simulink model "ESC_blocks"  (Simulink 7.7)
settings: Solver=ode45  StartTime=0.0  StopTime=10.0  RelTol=1e-3
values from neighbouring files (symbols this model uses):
  stepsize = 0.001    [sim_run_multi.m]    (also in sim_run_uni.m)
  x0 = [0;0]    [sim_run_multi.m]    (also in sim_run_uni.m = 0)
undefined symbols (not defined in the file or in its folder): adaptive_sampling, approx, nn, perturb, sm_periodic, vel_init_adap

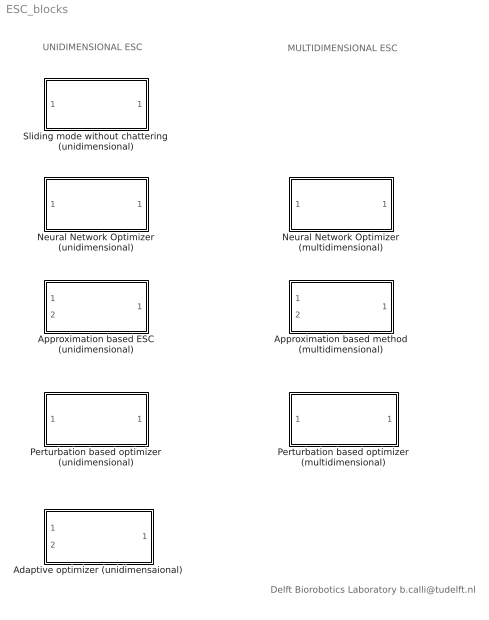
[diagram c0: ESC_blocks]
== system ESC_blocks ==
  note: UNIDIMENSIONAL ESC
  note: MULTIDIMENSIONAL ESC
  note: Delft Biorobotics Laboratory b.calli@tudelft.nl
  Adaptive optimizer (unidimensaional) : Subsystem  mask{adaptive_sampling=adaptive_sampling, vel_init=vel_init_adap, stepsize=stepsize, data_size=10, x0=x0}
      mask prompts: adaptive_sampling "Sampling (cycle)"; vel_init "Initial Velocity (while collecting initial data points)"; stepsize "Step size"; data_size "Data size"; x0 "Initial position"
  Approximation based ESC (unidimensional) : Subsystem  mask{K_grad=approx.K_grad, sampling=approx.sampling, data_size=approx.data_size, poly_degree=approx.poly_degree, vel_init=approx.vel_init, lpf_constant=approx.filter_constant}
      mask prompts: data_size "Data size"; poly_degree "Poly degree"; vel_init "Initial velocity"; lpf_constant "Filter Constant"
  Approximation based method (multidimensional) : Subsystem  mask{K_grad=approx.K_grad, sampling=approx.sampling, data_size=approx.data_size, vel_init=approx.vel_init, lpf_constant=approx.filter_constant}
      mask prompts: K_grad "Gain"; data_size "Data size"; vel_init "Initial velocity"; lpf_constant "Low pass filter constant"
  Neural Network Optimizer (multidimensional) : Subsystem  mask{M=nn.M, A=nn.A, B=nn.B, ddelta1=nn.ddelta1, ddelta2=nn.ddelta2, ddelta3=nn.ddelta3, delta=nn.delta, mpd_init=nn.mpd_init}
      mask prompts: ddelta1 "Direction 1 delta"; ddelta2 "Direction 2 delta"; ddelta3 "Direction 3 delta"; mpd_init "Minimum Peak Detector initial value"
  Neural Network Optimizer (unidimensional) : Subsystem  mask{M=nn.M, A=nn.A, B=nn.B, ddelta=nn.ddelta, delta=nn.delta, mpd_init=nn.mpd_init}
      mask prompts: mpd_init "Minimum peak detector initial value"
  Perturbation based optimizer (multidimensional) : Subsystem  mask{corr_gain=perturb.corr_gain, low_pass_pole=perturb.low_pass_pole, high_pass_pole=perturb.high_pass_pole, sine_amp=perturb.sine_amp, sine_freq=perturb.sine_freq, sine_phase=perturb.sine_phase, comp_zero=perturb.comp_zero, comp_pole=perturb.comp_pole}
      mask prompts: corr_gain "Correction gain"; low_pass_pole "Low Pass Filter pole"; high_pass_pole "High Pass Filter pole"; sine_amp "Sinus amplitude"; sine_freq "Sinus frequency"; sine_phase "Sinus phase"; comp_zero "Compensator zero"; comp_pole "Compensator pole"
  Perturbation based optimizer (unidimensional) : Subsystem  mask{high_pass_pole=perturb.high_pass_pole, sine_amp=perturb.sine_amp, sine_freq=perturb.sine_freq, low_pass_pole=perturb.low_pass_pole, corr_gain=perturb.corr_gain, comp_zero=perturb.comp_zero, comp_pole=perturb.comp_pole}
      mask prompts: high_pass_pole "High Pass Filter Pole"; sine_amp "Perturbation Signal Amplitude"; sine_freq "Perturbation Signal Frequency"; low_pass_pole "Low Pass Filter Pole"; corr_gain "Correction Gain"; comp_zero "Compensator Zero"; comp_pole "Compensator Pole"
  Sliding mode without chattering (unidimensional) : Subsystem  mask{alpha=sm_periodic.alpha, rho=sm_periodic.rho, k=sm_periodic.k, g_init=sm_periodic.g_init}
      mask prompts: g_init "initial g"

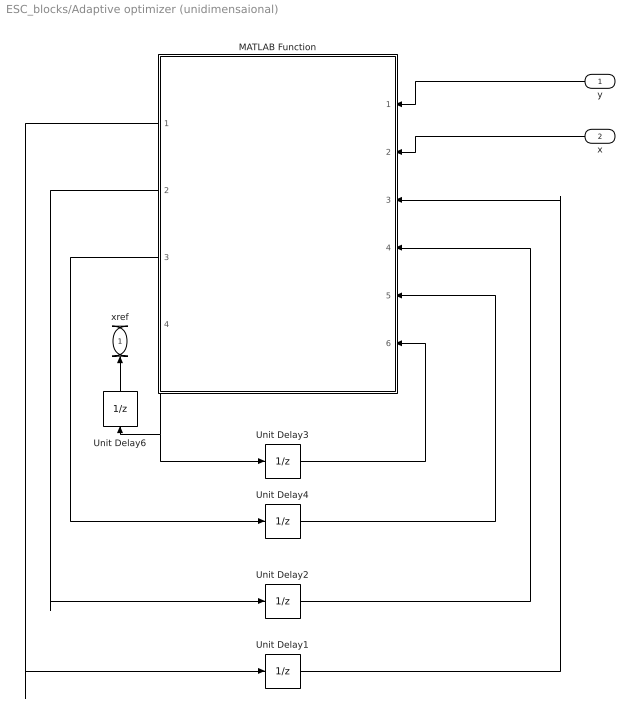
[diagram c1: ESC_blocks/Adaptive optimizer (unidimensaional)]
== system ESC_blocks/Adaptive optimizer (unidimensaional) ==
  y : Inport
  x : Inport  Port=2
  MATLAB Function : Stateflow chart  TreatAsAtomicUnit=on
  Unit Delay1 : UnitDelay  SampleTime=-1
  Unit Delay2 : UnitDelay  X0=zeros(data_size,3)  SampleTime=-1
  Unit Delay3 : UnitDelay  SampleTime=-1
  Unit Delay4 : UnitDelay  X0=zeros(data_size,1)  SampleTime=-1
  Unit Delay6 : UnitDelay  X0=x0  SampleTime=-1
  xref : Outport
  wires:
  y/1 -> MATLAB Function/1(y_data_in)
  MATLAB Function/4(x_ref) -> Unit Delay3/1, Unit Delay6/1
  Unit Delay3/1 -> MATLAB Function/6(x_ref_in)
  MATLAB Function/1(sample_out) -> Unit Delay1/1
  Unit Delay1/1 -> MATLAB Function/3(sample)
  MATLAB Function/2(phi_data_out) -> Unit Delay2/1
  MATLAB Function/3(y_array_out) -> Unit Delay4/1
  Unit Delay4/1 -> MATLAB Function/5(y_array)
  Unit Delay6/1 -> xref/1
  Unit Delay2/1 -> MATLAB Function/4(phi_data)
  x/1 -> MATLAB Function/2(x_in)

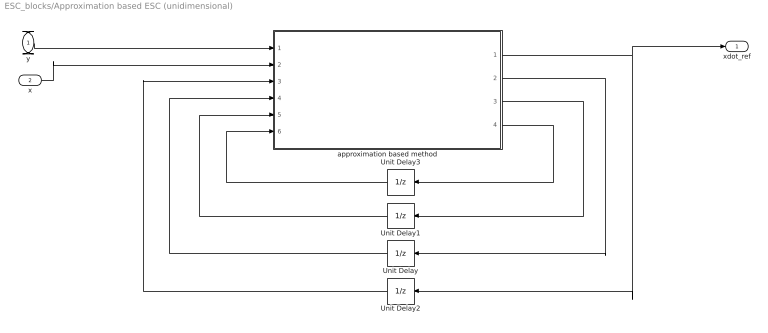
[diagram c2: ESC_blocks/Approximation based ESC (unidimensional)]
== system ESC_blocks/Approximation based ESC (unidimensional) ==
  y : Inport
  x : Inport  Port=2
  Unit Delay : UnitDelay  X0=zeros(1,data_size)  SampleTime=-1
  Unit Delay1 : UnitDelay  X0=zeros(1,data_size)  SampleTime=-1
  Unit Delay2 : UnitDelay  SampleTime=-1
  Unit Delay3 : UnitDelay  SampleTime=-1
  approximation based method : Stateflow chart  TreatAsAtomicUnit=on
  xdot_ref : Outport
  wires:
  approximation based method/2(x_data_arr_out) -> Unit Delay/1
  Unit Delay/1 -> approximation based method/4(x_data_arr)
  approximation based method/3(y_data_arr_out) -> Unit Delay1/1
  Unit Delay1/1 -> approximation based method/5(y_data_arr)
  y/1 -> approximation based method/1(y_data_in)
  x/1 -> approximation based method/2(x_data_in)
  approximation based method/1(xdot_ref) -> Unit Delay2/1, xdot_ref/1
  approximation based method/4(sample_out) -> Unit Delay3/1
  Unit Delay2/1 -> approximation based method/3(xdot_ref_in)
  Unit Delay3/1 -> approximation based method/6(sample)

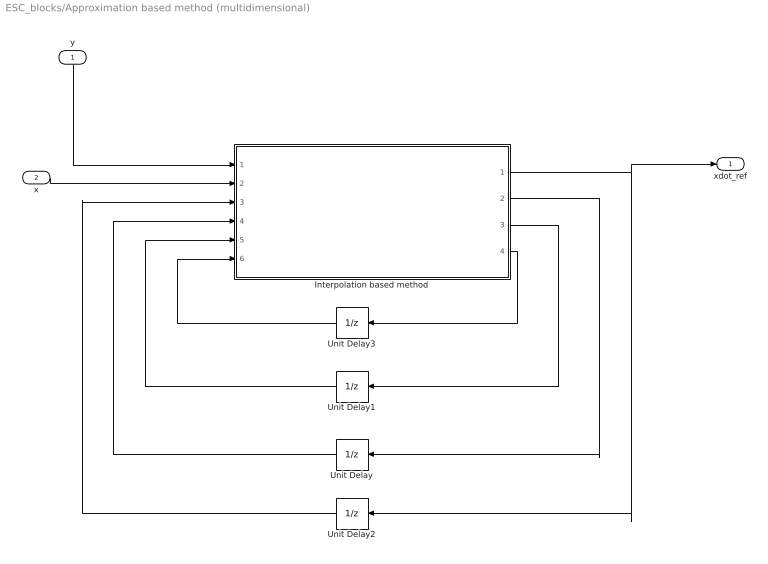
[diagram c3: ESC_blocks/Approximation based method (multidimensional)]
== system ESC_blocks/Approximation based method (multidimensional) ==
  y : Inport
  x : Inport  Port=2
  Interpolation based method : Stateflow chart  TreatAsAtomicUnit=on
  Unit Delay : UnitDelay  X0=[zeros(1,data_size);zeros(1,data_size)]  SampleTime=-1
  Unit Delay1 : UnitDelay  X0=zeros(1,data_size)  SampleTime=-1
  Unit Delay2 : UnitDelay  X0=[0;0]  SampleTime=-1
  Unit Delay3 : UnitDelay  SampleTime=-1
  xdot_ref : Outport
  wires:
  Unit Delay/1 -> Interpolation based method/4(x_data)
  Unit Delay1/1 -> Interpolation based method/5(y_data)
  y/1 -> Interpolation based method/1(y_data_in)
  x/1 -> Interpolation based method/2(x_data_in)
  Unit Delay2/1 -> Interpolation based method/3(xdot_ref_in)
  Unit Delay3/1 -> Interpolation based method/6(sample)
  Interpolation based method/4(sample_out) -> Unit Delay3/1
  Interpolation based method/3(y_data_out) -> Unit Delay1/1
  Interpolation based method/2(x_data_out) -> Unit Delay/1
  Interpolation based method/1(xdot_ref) -> Unit Delay2/1, xdot_ref/1

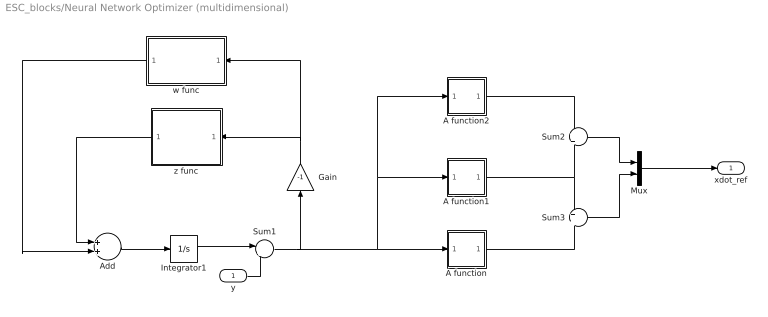
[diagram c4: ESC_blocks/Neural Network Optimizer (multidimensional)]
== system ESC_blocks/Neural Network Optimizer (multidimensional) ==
  y : Inport
  A function : Subsystem
  A function1 : Subsystem
  A function2 : Subsystem
  Add : Sum
  Gain : Gain  Gain=-1
  Integrator1 : Integrator  InitialCondition=mpd_init
  Mux : Mux  Inputs=2
  Sum1 : Sum  Inputs=|+-
  Sum2 : Sum  Inputs=+|+
  Sum3 : Sum  Inputs=+|+
  w func : Subsystem
  z func : Subsystem
  xdot_ref : Outport
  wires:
  Sum1/1 -> Gain/1, A function/1(e), A function1/1(e), A function2/1(e)
  Gain/1 -> w func/1(e_minus), z func/1(e_minus)
  w func/1(w) -> Add/2
  z func/1(z) -> Add/1
  Add/1 -> Integrator1/1
  Integrator1/1 -> Sum1/1
  A function2/1(xdot) -> Sum2/1
  A function1/1(xdot) -> Sum2/2, Sum3/1
  A function/1(xdot) -> Sum3/2
  Sum2/1 -> Mux/1
  Sum3/1 -> Mux/2
  Mux/1 -> xdot_ref/1
  y/1 -> Sum1/2

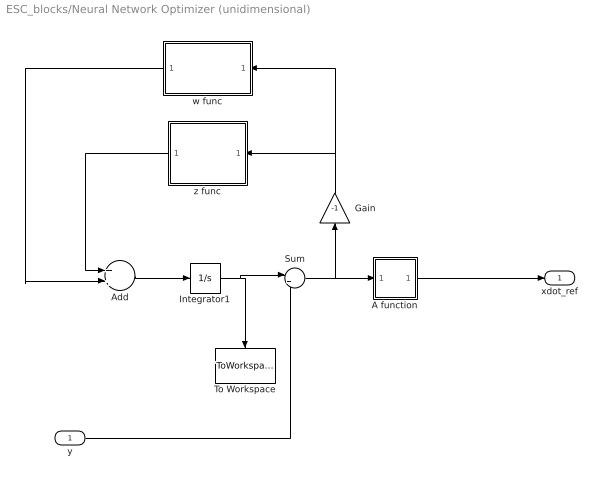
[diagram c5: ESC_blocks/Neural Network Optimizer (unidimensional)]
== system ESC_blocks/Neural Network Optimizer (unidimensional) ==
  y : Inport
  A function : Subsystem
  Add : Sum
  Gain : Gain  Gain=-1
  Integrator1 : Integrator  InitialCondition=mpd_init
  Sum : Sum  Inputs=|+-
  To Workspace : ToWorkspace  VariableName=yd_out  SampleTime=-1  SaveFormat=Structure With Time
  w func : Subsystem
  z func : Subsystem
  xdot_ref : Outport
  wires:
  Sum/1 -> Gain/1, A function/1(e)
  Gain/1 -> w func/1(e_minus), z func/1(e_minus)
  w func/1(w) -> Add/2
  z func/1(z) -> Add/1
  Add/1 -> Integrator1/1
  Integrator1/1 -> Sum/1, To Workspace/1
  A function/1(xdot) -> xdot_ref/1
  y/1 -> Sum/2

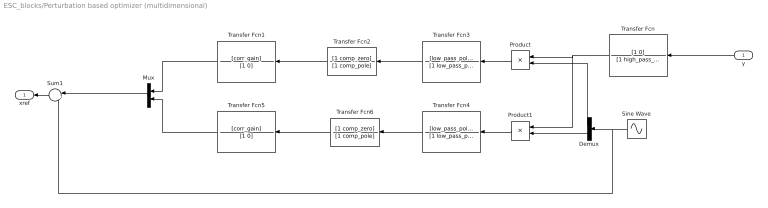
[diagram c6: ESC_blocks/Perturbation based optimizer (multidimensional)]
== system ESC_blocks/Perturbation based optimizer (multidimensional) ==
  y : Inport
  Demux : Demux  Outputs=2
  Mux : Mux  Inputs=2
  Product : Product  Multiplication=Matrix(*)
  Product1 : Product  Multiplication=Matrix(*)
  Sine Wave : Sin  Amplitude=[sine_amp sine_amp]  Frequency=[sine_freq sine_freq]  Phase=[0 sine_phase]  SampleTime=0
  Sum1 : Sum  Inputs=|++
  Transfer Fcn : TransferFcn  Numerator=[1 0]  Denominator=[1 high_pass_pole]
  Transfer Fcn1 : TransferFcn  Numerator=[corr_gain]  Denominator=[1 0]
  Transfer Fcn2 : TransferFcn  Numerator=[1 comp_zero]  Denominator=[1 comp_pole]
  Transfer Fcn3 : TransferFcn  Numerator=[low_pass_pole]  Denominator=[1 low_pass_pole]
  Transfer Fcn4 : TransferFcn  Numerator=[low_pass_pole]  Denominator=[1 low_pass_pole]
  Transfer Fcn5 : TransferFcn  Numerator=[corr_gain]  Denominator=[1 0]
  Transfer Fcn6 : TransferFcn  Numerator=[1 comp_zero]  Denominator=[1 comp_pole]
  xref : Outport
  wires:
  y/1 -> Transfer Fcn/1
  Sum1/1 -> xref/1
  Transfer Fcn/1 -> Product/1, Product1/1
  Sine Wave/1 -> Demux/1, Sum1/2
  Demux/1 -> Product/2
  Demux/2 -> Product1/2
  Product/1 -> Transfer Fcn3/1
  Product1/1 -> Transfer Fcn4/1
  Transfer Fcn3/1 -> Transfer Fcn2/1
  Transfer Fcn4/1 -> Transfer Fcn6/1
  Transfer Fcn1/1 -> Mux/1
  Transfer Fcn5/1 -> Mux/2
  Mux/1 -> Sum1/1
  Transfer Fcn2/1 -> Transfer Fcn1/1
  Transfer Fcn6/1 -> Transfer Fcn5/1

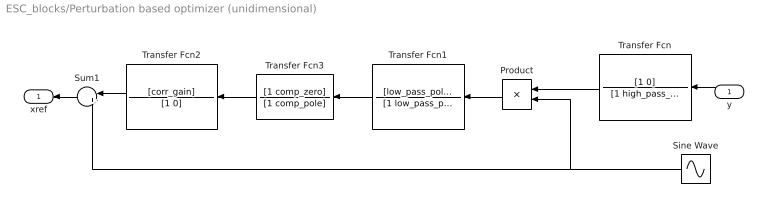
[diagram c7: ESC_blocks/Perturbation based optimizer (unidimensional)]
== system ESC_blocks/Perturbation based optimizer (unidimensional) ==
  y : Inport
  Product : Product
  Sine Wave : Sin  Amplitude=sine_amp  Frequency=sine_freq  SampleTime=0
  Sum1 : Sum  Inputs=|++
  Transfer Fcn : TransferFcn  Numerator=[1 0]  Denominator=[1 high_pass_pole]
  Transfer Fcn1 : TransferFcn  Numerator=[low_pass_pole]  Denominator=[1 low_pass_pole]
  Transfer Fcn2 : TransferFcn  Numerator=[corr_gain]  Denominator=[1 0]
  Transfer Fcn3 : TransferFcn  Numerator=[1 comp_zero]  Denominator=[1 comp_pole]
  xref : Outport
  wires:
  Transfer Fcn/1 -> Product/1
  Sine Wave/1 -> Product/2, Sum1/2
  Product/1 -> Transfer Fcn1/1
  Transfer Fcn1/1 -> Transfer Fcn3/1
  Transfer Fcn2/1 -> Sum1/1
  y/1 -> Transfer Fcn/1
  Sum1/1 -> xref/1
  Transfer Fcn3/1 -> Transfer Fcn2/1

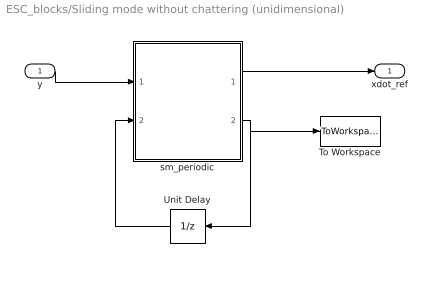
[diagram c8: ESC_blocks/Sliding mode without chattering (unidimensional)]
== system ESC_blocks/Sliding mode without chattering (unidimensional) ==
  y : Inport
  To Workspace : ToWorkspace  VariableName=g_sm_out  SampleTime=-1  SaveFormat=Structure With Time
  Unit Delay : UnitDelay  X0=g_init  SampleTime=-1
  sm_periodic : Stateflow chart  TreatAsAtomicUnit=on
  xdot_ref : Outport
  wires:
  y/1 -> sm_periodic/1(y)
  sm_periodic/1(u) -> xdot_ref/1
  sm_periodic/2(g_out) -> Unit Delay/1, To Workspace/1
  Unit Delay/1 -> sm_periodic/2(g_in)

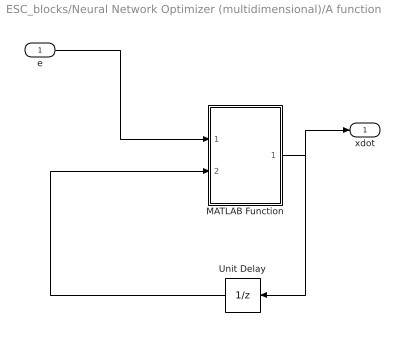
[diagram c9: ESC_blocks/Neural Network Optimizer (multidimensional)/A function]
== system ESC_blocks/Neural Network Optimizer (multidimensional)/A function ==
  e : Inport
  MATLAB Function : Stateflow chart  TreatAsAtomicUnit=on
  Unit Delay : UnitDelay  X0=A  SampleTime=-1
  xdot : Outport
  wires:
  Unit Delay/1 -> MATLAB Function/2(state_pre)
  MATLAB Function/1(xdot) -> xdot/1, Unit Delay/1
  e/1 -> MATLAB Function/1(e)

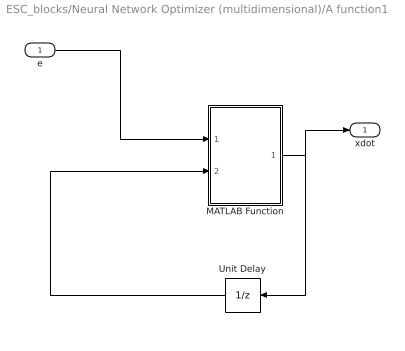
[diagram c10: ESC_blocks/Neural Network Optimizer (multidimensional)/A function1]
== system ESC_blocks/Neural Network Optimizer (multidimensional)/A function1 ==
  e : Inport
  MATLAB Function : Stateflow chart  TreatAsAtomicUnit=on
  Unit Delay : UnitDelay  SampleTime=-1
  xdot : Outport
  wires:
  e/1 -> MATLAB Function/1(e)
  MATLAB Function/1(xdot) -> Unit Delay/1, xdot/1
  Unit Delay/1 -> MATLAB Function/2(state_pre)

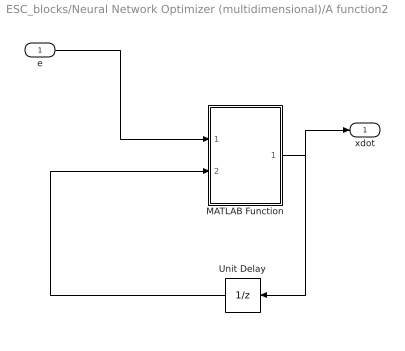
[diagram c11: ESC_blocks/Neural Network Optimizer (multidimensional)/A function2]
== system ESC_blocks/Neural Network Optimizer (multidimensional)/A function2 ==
  e : Inport
  MATLAB Function : Stateflow chart  TreatAsAtomicUnit=on
  Unit Delay : UnitDelay  SampleTime=-1
  xdot : Outport
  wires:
  Unit Delay/1 -> MATLAB Function/2(state_pre)
  MATLAB Function/1(xdot) -> xdot/1, Unit Delay/1
  e/1 -> MATLAB Function/1(e)

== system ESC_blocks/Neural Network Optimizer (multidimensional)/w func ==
  e_minus : Inport
  MATLAB Function2 : Stateflow chart  TreatAsAtomicUnit=on
  Unit Delay : UnitDelay  SampleTime=-1
  w : Outport
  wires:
  e_minus/1 -> MATLAB Function2/1(e_minus)
  MATLAB Function2/1(w) -> w/1, Unit Delay/1
  Unit Delay/1 -> MATLAB Function2/2(state_pre)

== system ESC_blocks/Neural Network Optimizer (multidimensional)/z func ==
  e_minus : Inport
  MATLAB Function1 : Stateflow chart  TreatAsAtomicUnit=on
  z : Outport
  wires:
  e_minus/1 -> MATLAB Function1/1(e_minus)
  MATLAB Function1/1(z) -> z/1

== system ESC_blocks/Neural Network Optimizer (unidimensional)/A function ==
  e : Inport
  MATLAB Function : Stateflow chart  TreatAsAtomicUnit=on
  Unit Delay : UnitDelay  X0=A  SampleTime=-1
  xdot : Outport
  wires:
  Unit Delay/1 -> MATLAB Function/2(x_dot_pre)
  MATLAB Function/1(xdot) -> xdot/1, Unit Delay/1
  e/1 -> MATLAB Function/1(e)

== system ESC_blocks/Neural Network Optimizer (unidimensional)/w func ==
  e_minus : Inport
  MATLAB Function2 : Stateflow chart  TreatAsAtomicUnit=on
  Unit Delay : UnitDelay  SampleTime=-1
  w : Outport
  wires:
  e_minus/1 -> MATLAB Function2/1(e_minus)
  Unit Delay/1 -> MATLAB Function2/2(w_pre)
  MATLAB Function2/1(w) -> w/1, Unit Delay/1

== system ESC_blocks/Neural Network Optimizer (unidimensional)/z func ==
  e_minus : Inport
  MATLAB Function1 : Stateflow chart  TreatAsAtomicUnit=on
  z : Outport
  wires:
  e_minus/1 -> MATLAB Function1/1(e_minus)
  MATLAB Function1/1(z) -> z/1

== matlab function Neural Network Optimizer
(unidimensional)/A function/MATLAB Function ==
function xdot = nn_ESC(e,x_dot_pre,A,ddelta)
%#codegen

if( e<-ddelta )
    xdot = -A;
elseif(e>ddelta)
    xdot = A;
else
    xdot = x_dot_pre;
end

end

== matlab function Approximation based ESC
(unidimensional)/approximation based method ==
function [xdot_ref,x_data_arr_out,y_data_arr_out, sample_out] = approx_based_method(y_data_in, x_data_in, xdot_ref_in, x_data_arr, y_data_arr,K_grad, sample, sampling, poly_degree, data_size, vel_init, lpf_constant)
%#codegen
if(mod(sample,sampling) == 0)
    sample_out = sample+1;
    x_data_arr = circshift(x_data_arr,1);
    y_data_arr = circshift(y_data_arr,1);
    x_data_arr(1) = x_data_in;
    y_data_arr(1) = y_data_in;
    
    V = zeros(data_size,poly_degree+1);

    % forming the vandermonde matrix 
    for i=1:data_size
        for j=1:poly_degree+1
            V(i,j) = x_data_arr(i)^(poly_degree-j+1);
        end
    end
   
    c = pinv(V)*y_data_arr;     % calculating coefficients
    x = x_data_arr(1);
    
    % calculating gradient
    grad_val = 0; 
    for i = 1:poly_degree
        grad_val = grad_val+c(i)*(poly_degree+1-i)*x.^(poly_degree-i);
    end
    
    
    if (sample<sampling*data_size)      % collecting first set for approximation with a constant velocity
        xdot_ref = vel_init;
    else                                % calculating velocity references otherwise
        xdot_ref = -K_grad*grad_val;
        if (xdot_ref~=xdot_ref)         % if the result of the approximation is NAN because of an ill-poised data set, keep the previous the velocity reference.
            xdot_ref = xdot_ref_in;
        end
    end
    
    % apply lowpass filtering for output
    if(xdot_ref~=vel_init)
        xdot_ref = lpf_constant * xdot_ref + ( 1.0 - lpf_constant ) * xdot_ref_in;
    end
    
    x_data_arr_out = x_data_arr;
    y_data_arr_out = y_data_arr;
else
    sample_out = sample+1;
    x_data_arr_out = x_data_arr;
    y_data_arr_out = y_data_arr;
    xdot_ref = xdot_ref_in;
end

== matlab function Neural Network Optimizer
(unidimensional)/z func/MATLAB Function1 ==
function z = zfunc(e_minus,M)
%#codegen
if(e_minus>0)
    z = 0;
else
    z = -M;
end
end

== matlab function Neural Network Optimizer
(unidimensional)/w func/MATLAB Function2 ==
function w = wfunc(e_minus,w_pre,B,delta)
%#codegen
if(e_minus<-delta)
    w = 0;
elseif (e_minus>delta)
    w = B;
else
    w = w_pre;
end
end

== matlab function Neural Network Optimizer
(multidimensional)/A function1/MATLAB Function ==
function xdot = fnc1(e,state_pre,A,ddelta2)
%#codegen

if( e<-ddelta2 )
    xdot = 0;
elseif(e>ddelta2)
    xdot = A;
else
    xdot = state_pre;
end

end

== matlab function Neural Network Optimizer
(multidimensional)/A function/MATLAB Function ==
function xdot = fnc(e,state_pre,A,ddelta1)
%#codegen

if( e<-ddelta1 )
    xdot = -A;
elseif(e>ddelta1)
    xdot = A;
else
    xdot = state_pre;
end

end

== matlab function Approximation based method
(multidimensional)/Interpolation based
method ==
function [xdot_ref,x_data_out,y_data_out, sample_out] = interpolation_based_method(y_data_in, x_data_in, xdot_ref_in, x_data, y_data,K_grad, sample, sampling, data_size, vel_init, lpf_constant)
%#codegen
if(mod(sample,sampling) == 0 )
    sample_out = sample+1;
    x1_data = x_data(1,:);
    x2_data = x_data(2,:);
    x1_data = circshift(x1_data,[0,1]);
    x2_data = circshift(x2_data,[0,1]);
    y_data = circshift(y_data,1);
    x1_data(1) = x_data_in(1,1);
    x2_data(1) = x_data_in(2,1);
    y_data(1) = y_data_in;
    
    V = zeros(data_size,4);
    
    for i=1:data_size
        V(i,:) = [x1_data(i)*x2_data(i) x1_data(i) x2_data(i) 1];
    end

    c = pinv(V)*y_data;
    x = [x1_data(1);x2_data(1)];
    grad_val = [c(1)*x(2)+c(2);
                c(1)*x(1)+c(3)];
    %grad_val = grad_val./norm(grad_val,1);

    if (sample<sampling*data_size)
        xdot_ref = [vel_init;vel_init];
    else
        xdot_ref = -K_grad*grad_val;
        
        if (xdot_ref(1)~=xdot_ref(1) || xdot_ref(2)~=xdot_ref(2))
            xdot_ref = [0;0];
        end
    end

    if(xdot_ref(1)==vel_init && xdot_ref(2)==vel_init)
    else
        xdot_ref(1) = lpf_constant * xdot_ref(1) + ( 1.0 - lpf_constant ) * xdot_ref_in(1);
        xdot_ref(2) = lpf_constant * xdot_ref(2) + ( 1.0 - lpf_constant ) * xdot_ref_in(2);
    end
    
    x_data_out = [x1_data; x2_data];
    y_data_out = y_data;
else
    sample_out = sample+1;
    x_data_out = x_data;
    y_data_out = y_data;
    xdot_ref = xdot_ref_in;
end

== matlab function Sliding mode without chattering
(unidimensional)/sm_periodic ==
function [u,g_out]  = sm_periodic(y,g_in,alpha, k, rho)
%#codegen

g_out = g_in-rho;
s = y-g_out;

u = k*sign(sin(pi/alpha*s));

== matlab function Neural Network Optimizer
(multidimensional)/A function2/MATLAB Function ==
function xdot = fnc3(e,state_pre,A,ddelta3)
%#codegen

if( e<-ddelta3 )
    xdot = -2*A;
elseif(e>ddelta3)
    xdot = 0;
else
    xdot = state_pre;
end

end

== matlab function Neural Network Optimizer
(multidimensional)/w func/MATLAB Function2 ==
function w = wfunc(e_minus,state_pre,B,delta)
%#codegen
if(e_minus<-delta)
    w = 0;
elseif (e_minus>delta)
    w = B;
else
    w = state_pre;
end
end

== matlab function Neural Network Optimizer
(multidimensional)/z func/MATLAB Function1 ==
function z = zfunc(e_minus,M)
%#codegen
if(e_minus>0)
    z = 0;
else
    z = -M;
end
end

== matlab function Adaptive optimizer
(unidimensaional)/MATLAB Function ==
function [sample_out,phi_data_out,y_array_out,x_ref] = adaptive_esc(y_data_in,x_in,sample, phi_data, y_array,x_ref_in,adaptive_sampling, vel_init, stepsize, data_size)
%#codegen

if(mod(sample,adaptive_sampling) == 0)
    
    phi_data = circshift(phi_data,1);
    y_array = circshift(y_array,1);
    phi_data(1,1) = 1;
    phi_data(1,2) = x_in;
    phi_data(1,3) = x_in^2;
    y_array(1) = y_data_in;
    if (sample<=adaptive_sampling*data_size+100)
        x_ref = x_ref_in-vel_init*stepsize;
    else
        params = pinv(phi_data)*y_array;
        x_ref = -params(2)/(2*params(3));
    end
    phi_data_out = phi_data;
    y_array_out = y_array;
    sample_out = sample+1;
else
    sample_out = sample+1;
    phi_data_out = phi_data;
    y_array_out = y_array;
    x_ref = x_ref_in;
end
